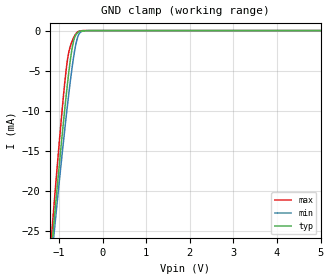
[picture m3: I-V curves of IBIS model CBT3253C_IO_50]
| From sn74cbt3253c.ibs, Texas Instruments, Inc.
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[Model]   CBT3253C_IO_50
Model_type  Terminator
| variable   typ   min   max
C_comp   13.68pF   10.66pF   19.31pF
| C_tri-state   13.68pF   10.66pF   19.31pF
[Temperature Range]   40   100   -40
| Ambient temperature   25   85   -40
[Voltage range]   5   4.5   5.5
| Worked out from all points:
|   GND clamp passes 1 mA (typ) near -0.65 V on its own axis
[GND Clamp]
| CBT3253C_IO_50
|   Voltage   I(typ)   I(min)   I(max)
-5V       -286.9mA   -267.5mA   -309.2mA
-1.155V   -26.34mA   -27.64mA   -24.51mA
-1.12V    -24.23mA   -25.7mA    -22.17mA
-1.085V   -22.14mA   -23.78mA   -19.85mA
-925mV    -12.91mA   -15.26mA   -9.733mA
-815mV    -7.1mA     -9.759mA   -4.012mA
-760mV    -4.528mA   -7.199mA   -2.356mA
-680mV    -1.666mA   -3.864mA   -1.075mA
-610mV    -508.3uA   -1.615mA   -383.4uA
-545mV    -149.1uA   -476.8uA   -90.44uA
-310mV    -1.145uA   -5.133uA   -22.33nA
5V        1.01nA     2.646nA    473.6pA
